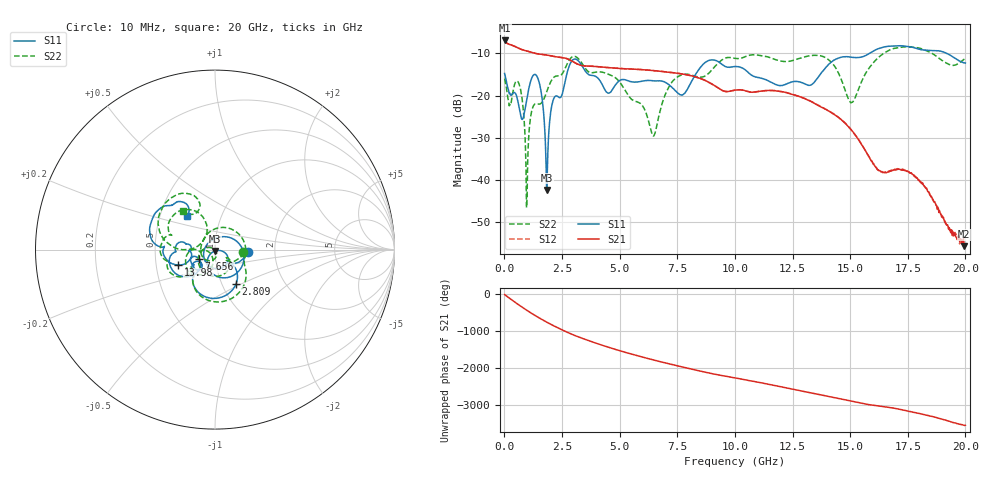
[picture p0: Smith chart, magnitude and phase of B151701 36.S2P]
!  2-Port S-parameters saved by WinCal
! VAR MeasName=S-Parameters (CALIBRATED_DATA) read from VNA (N5244A)
! VAR MeasDate=2015-12-24 19:13:34
! VAR NAME=B151701 36
! VAR FILENAME=B151701 36.S2P
! VAR DATE=2015-12-24 19:13:34
! VAR PHYS_PORTS=1,3
# Hz S DB R 50
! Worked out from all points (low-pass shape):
!   801 points, 10 MHz to 20 GHz, reference 50 ohm
!   highest |S21| = -6.91 dB at 10 MHz (marker M1); lowest = -55.6 dB at 19.95 GHz (marker M2)
!   |S21| within 3 dB of the highest: start of sweep to 1.289 GHz
!   lowest |S11| = -42.3 dB at 1.834 GHz (marker M3), VSWR 1.02, Z = 50 - j0.765 ohm
!   |S11| at or under -10 dB: start of sweep to 15.83 GHz; 19.19 GHz to end of sweep
!   |S22| runs from -46.5 to -8.4 dB; largest |S21 - S12| = 0.0014
!   S11 on the Smith chart (normalised r, x): 10 MHz: 1.45, -0.05; 2.809 GHz: 1.17, -0.47; 7.656 GHz: 0.83, -0.09; 13.98 GHz: 0.65, -0.12; 20 GHz: 0.69, +0.27
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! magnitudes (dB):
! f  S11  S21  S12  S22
! 10 MHz  -14.7  -6.9  -6.9  -16.0
! 659.7 MHz  -23.5  -8.9  -8.9  -17.6
! 984.5 MHz  -20.4  -9.4  -9.4  -44.3
! 1.184 GHz  -15.9  -9.8  -9.7  -23.6
! 1.459 GHz  -16.0  -10.1  -10.1  -21.9
! 1.834 GHz  -42.3  -10.4  -10.4  -19.1
! 2.109 GHz  -21.2  -10.6  -10.7  -15.9
! 2.809 GHz  -13.0  -11.4  -11.4  -11.6
! 3.358 GHz  -12.8  -12.9  -12.9  -12.3
! 4.508 GHz  -19.4  -13.3  -13.3  -14.9
! 6.432 GHz  -16.4  -14.0  -14.0  -29.4
! 6.682 GHz  -16.5  -14.2  -14.2  -25.3
! 7.656 GHz  -19.8  -14.8  -14.8  -15.1
! 8.806 GHz  -11.8  -16.6  -16.6  -15.0
! 10.01 GHz  -13.1  -18.7  -18.6  -11.2
! 13.35 GHz  -17.3  -21.5  -21.5  -10.5
! 13.98 GHz  -13.1  -23.3  -23.3  -11.1
! 15.05 GHz  -10.9  -28.1  -28.2  -21.6
! 16.68 GHz  -8.3  -37.9  -37.9  -9.3
! 17.8 GHz  -8.7  -39.0  -39.0  -8.6
! 19.95 GHz  -12.2  -55.6  -55.5  -11.3
! 20 GHz  -12.3  -55.4  -55.6  -11.1
